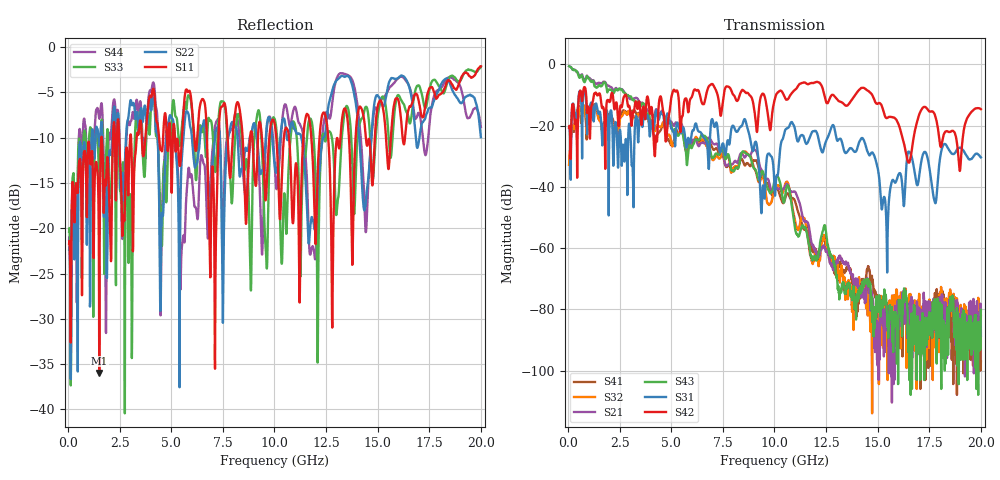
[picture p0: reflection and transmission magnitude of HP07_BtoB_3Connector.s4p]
# MHz S MA R 50.00
! FREQ  S11  S12  S13  S14
!  S21  S22  S23  S24
!  S31  S32  S33  S34
!  S41  S42  S43  S44
!  MAG  ANG  MAG  ANG  MAG  ANG  MAG  ANG
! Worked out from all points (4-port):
!   1996 points, 50 MHz to 20 GHz, reference 50 ohm
!   strongest paths, dB at 50 MHz, 5.04 GHz, 10.03 GHz, 15.02 GHz, 20 GHz:
!     S42: -20.6, -9.7, -11.0, -12.7, -14.6
!     S31: -20.6, -21.1, -42.9, -34.6, -30.4
!     S43: -0.6, -21.3, -37.3, -78.0, -80.2
!     S21: -0.6, -19.3, -40.3, -93.2, -88.6
!     S32: -32.7, -26.6, -40.3, -80.6, -82.2
!     S41: -32.7, -26.5, -40.2, -76.6, -97.1
!   lowest |S11| = -36.0 dB at 1.51 GHz (marker M1), VSWR 1.03, Z = 49 + j1.24 ohm
!   |S11| at or under -10 dB: start of sweep to 1.613 GHz; 10.7 GHz to 11.4 GHz (695.3 MHz wide, 6.29 % of centre); 12.6 GHz to 13.2 GHz (593.6 MHz wide, 4.6 % of centre)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
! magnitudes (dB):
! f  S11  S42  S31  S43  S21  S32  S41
! 50 MHz  -21.7  -20.6  -20.6  -0.6  -0.6  -32.7  -32.7
! 1.51 GHz  -36.0  -9.4  -15.9  -6.7  -6.1  -18.2  -17.6
! 8.56 GHz  -15.9  -8.9  -17.9  -28.7  -30.4  -28.4  -33.0
! 9.42 GHz  -10.8  -9.6  -41.3  -34.9  -35.1  -36.5  -35.7
! 12.83 GHz  -24.0  -9.9  -19.8  -63.3  -66.9  -62.9  -66.0
! 15.45 GHz  -11.7  -17.5  -63.5  -80.6  -79.0  -87.3  -82.7
! 20 GHz  -2.1  -14.6  -30.4  -80.2  -88.6  -82.2  -97.1
